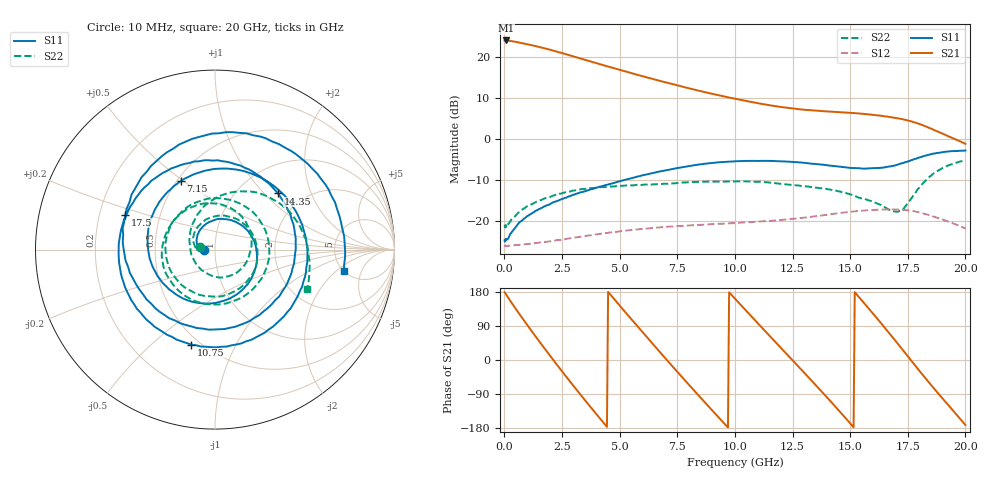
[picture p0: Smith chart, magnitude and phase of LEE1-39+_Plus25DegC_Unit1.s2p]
!Keysight Technologies,N5245A,MY52442000,A.10.65.23
!Date: Tuesday, November 25, 2025 21:52:59
!Correction: S11(Full 2 Port(1,2))
!S21(Full 2 Port(1,2))
!S12(Full 2 Port(1,2))
!S22(Full 2 Port(1,2))
!S2P File: Measurements: S11, S21, S12, S22:
!Deduct Board Loss
# Hz S  dB  R 50
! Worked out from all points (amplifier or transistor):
!   408 points, 10 MHz to 20 GHz, reference 50 ohm
!   highest |S21| = 24.0 dB at 60 MHz (marker M1)
!   |S21| within 3 dB of that: start of sweep to 2.459 GHz
!   unconditionally stable (mu >= 1): start of sweep to end of sweep
!   at 3.05 GHz: K = 1.04, MAG = 20.7 dB, |S12| = -23.9 dB
!   at 9.85 GHz: K = 1.30, MAG = 11.9 dB, |S12| = -20.4 dB
!   at 20 GHz: K = 2.42, MAG = 3.7 dB, |S12| = -21.8 dB
!   S11 on the Smith chart (normalised r, x): 10 MHz: 0.89, +0.00; 7.15 GHz: 0.52, +0.49; 10.75 GHz: 0.45, -0.68; 14.35 GHz: 1.51, +1.21; 17.5 GHz: 0.31, +0.17; 20 GHz: 5.01, -2.58
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1e7  -24.61 179.6  23.91 178.9  -25.91 0.3  -21.25 169.5
6e7  -24.25 -177.1  23.98 174.3  -25.84 -2.8  -21.31 -178.6
5e8  -21.29 177.3  23.63 134.4  -25.72 -23.6  -18.50 167.0
9e8  -19.13 157.3  23.18 100.0  -25.53 -44.0  -16.64 141.8
1.3e9  -17.67 134.4  22.68 66.6  -25.26 -64.3  -15.48 114.2
1.85e9  -16.05 101.3  21.91 21.7  -24.90 -92.8  -14.20 77.0
2.65e9  -14.26 51.3  20.67 -41.5  -24.29 -134.9  -12.91 22.6
3.35e9  -12.86 5.5  19.51 -95.1  -23.68 -173.3  -12.14 -24.9
3.95e9  -11.90 -33.5  18.54 -139.9  -23.15 153.2  -11.80 -65.2
4.5e9  -11.03 -69.8  17.64 179.8  -22.76 122.1  -11.54 -102.5
5.55e9  -9.41 -139.2  15.98 104.6  -22.05 61.3  -11.25 -173.5
6.7e9  -7.89 145.9  14.24 24.1  -21.45 -6.2  -10.96 109.0
7.15e9  -7.41 116.5  13.59 -6.9  -21.24 -32.9  -10.82 78.9
8.35e9  -6.24 40.6  11.88 -88.5  -20.87 -103.4  -10.40 2.1
1.005e10  -5.38 -62.0  9.78 158.8  -20.37 157.5  -10.27 -98.4
1.075e10  -5.27 -104.1  9.01 113.0  -20.11 116.6  -10.31 -135.8
1.215e10  -5.43 173.6  7.70 22.0  -19.56 35.0  -10.95 153.4
1.335e10  -5.94 103.3  7.00 -56.0  -18.87 -35.6  -11.63 98.5
1.435e10  -6.53 41.5  6.63 -122.5  -18.11 -96.3  -12.46 53.1
1.67e10  -6.63 -135.4  5.40 70.7  -17.09 110.2  -17.14 -112.5
1.75e10  -5.42 158.7  4.56 10.0  -17.29 54.0  -15.59 146.7
2e10  -2.75 -9.5  -1.16 -171.4  -21.76 -113.2  -5.06 -23.3
